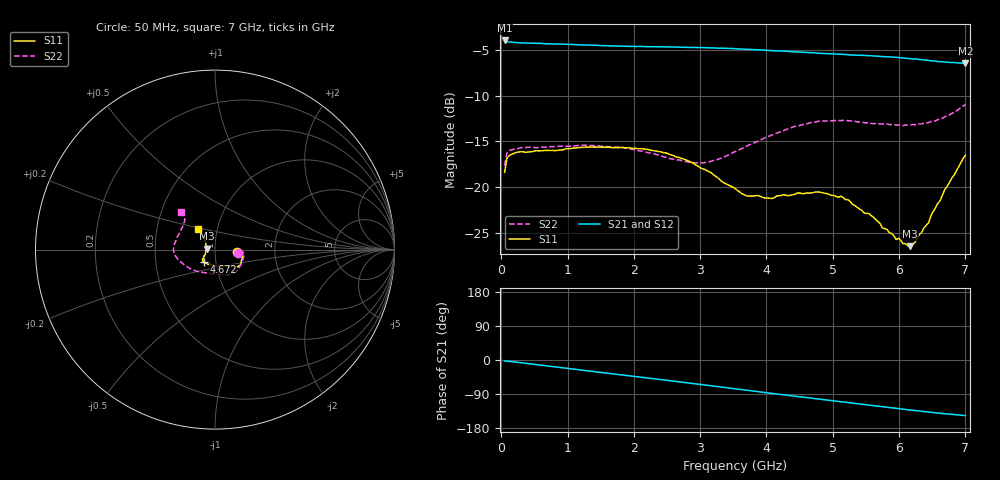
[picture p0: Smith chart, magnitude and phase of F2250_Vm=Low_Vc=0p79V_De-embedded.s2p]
! Integrated Device Technology
! Corporate Headquarters
! 6024 Silver Creek Valley Road
! San Jose, CA 95138  USA
! Phone:  1-408-284-8200
! Toll Free:  1-800-223-1366
! Webpage:  http://www.idt.com/
! Timing and RF Division
! 515 Groton Road, Suite 102
! Westford, MA 01886-6024
! Device:  F2250
! Description: Voltage Variable RF Attenuator
! Frequency:  50.0 -  6000.00 MHz
! Package:  3x3 mm Thin QFN Plastic Package: 16 pin
! Ports:  2 RF, 3 DC
!  Pin  1  = GND
!  Pin  2  = NC
!  Pin  3  = RF1  = Port 1
!  Pin  4  = NC
!  Pin  5  = GND
!  Pin  6  = GND
!  Pin  7  = GND
!  Pin  8  = GND
!  Pin  9  = NC
!  Pin 10  = RF2  = Port 2
!  Pin 11  = NC
!  Pin 12  = GND
!  Pin 13  = GND
!  Pin 14  = VCNTRL
!  Pin 15  = VDD
!  Pin 16  = VMODE
! Vcntrl:  0.790 Volts
! Vmode:  +0.000 Volts
! Vdd:  +3.30  Volts
! Current:  1.165 mA
! Data:  The device was measured on a the F2250 evaluation board which has
!  individual transmission lines to the RF pins.  Data was collected
!  using a calibrated network analyzer.  The evaluation board was
!  de-embedded using a TRL calibration technique.
!  The reference plane is the edge of the package pin.
! Misc:  SN 10
!  Action Tracker AT0258
! Date Measured:  2014-11-26
! Date:  2015-10-15  MJV
! Note:
!  Integrated Device Technology supplies this data as a sample of measured
!  data at the package pin for this product.  Your particular data for this
!  product may vary.
!  Data was taken at 25 degrees C.
!  Integrated Device Technology reserves the right to change this data at anytime.
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# GHz S dB R 50
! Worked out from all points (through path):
!   201 points, 50 MHz to 7 GHz, reference 50 ohm
!   highest |S21| = -3.95 dB at 50 MHz (marker M1); lowest = -6.5 dB at 7 GHz (marker M2)
!   group delay of S21, straight-line fit = 58.8 ps
!   lowest |S11| = -26.5 dB at 6.166 GHz (marker M3), VSWR 1.10, Z = 45.5 + j0.553 ohm
!   |S11| at or under -10 dB: start of sweep to end of sweep
!   |S22| runs from -17.6 to -11.0 dB; largest |S21 - S12| = 0.0015
!   S11 on the Smith chart (normalised r, x): 50 MHz: 1.27, -0.04; 4.672 GHz: 0.87, -0.12; 7 GHz: 0.80, +0.19
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0.05  -18.37 -6.8  -3.95 -2.6  -3.95 -2.6  -17.64 -7.6
0.08475  -16.85 -4.9  -4.08 -2.9  -4.09 -2.9  -16.27 -5.8
0.22375  -16.22 -6.9  -4.18 -5.7  -4.20 -5.7  -15.80 -9.6
1.2315  -15.65 -28.9  -4.45 -27.2  -4.45 -27.2  -15.43 -43.7
1.857  -15.69 -34.5  -4.57 -40.2  -4.58 -40.2  -15.69 -58.0
2.37825  -16.10 -37.1  -4.65 -51.0  -4.65 -51.0  -16.50 -70.6
3.0385  -18.00 -48.4  -4.74 -65.3  -4.73 -65.3  -17.36 -100.9
3.525  -20.15 -70.5  -4.85 -76.0  -4.87 -76.0  -16.12 -129.0
3.69875  -20.96 -82.1  -4.92 -79.8  -4.91 -79.8  -15.53 -137.6
4.081  -21.25 -107.2  -5.06 -88.1  -5.06 -88.1  -14.31 -154.5
4.67175  -20.65 -133.1  -5.29 -100.8  -5.29 -100.8  -12.94 -172.1
4.7065  -20.59 -134.0  -5.30 -101.5  -5.30 -101.5  -12.93 -172.9
5.22775  -21.37 -143.0  -5.52 -112.4  -5.52 -112.4  -12.73 175.4
5.61  -23.28 -149.3  -5.65 -120.4  -5.66 -120.4  -13.07 166.0
5.85325  -25.00 -160.7  -5.74 -125.3  -5.77 -125.4  -13.16 159.6
5.9575  -25.75 -167.7  -5.80 -127.5  -5.81 -127.6  -13.23 156.6
5.99225  -25.60 -170.8  -5.81 -128.3  -5.83 -128.3  -13.20 155.6
6.06175  -26.22 -176.1  -5.87 -129.7  -5.88 -129.7  -13.28 153.2
6.166  -26.47 172.7  -5.94 -131.8  -5.95 -131.8  -13.20 149.8
6.444  -23.92 143.1  -6.13 -137.4  -6.14 -137.4  -12.95 140.7
6.68725  -20.29 131.3  -6.32 -141.6  -6.33 -141.7  -12.29 134.1
7  -16.51 130.2  -6.46 -146.7  -6.47 -146.7  -10.97 131.7
